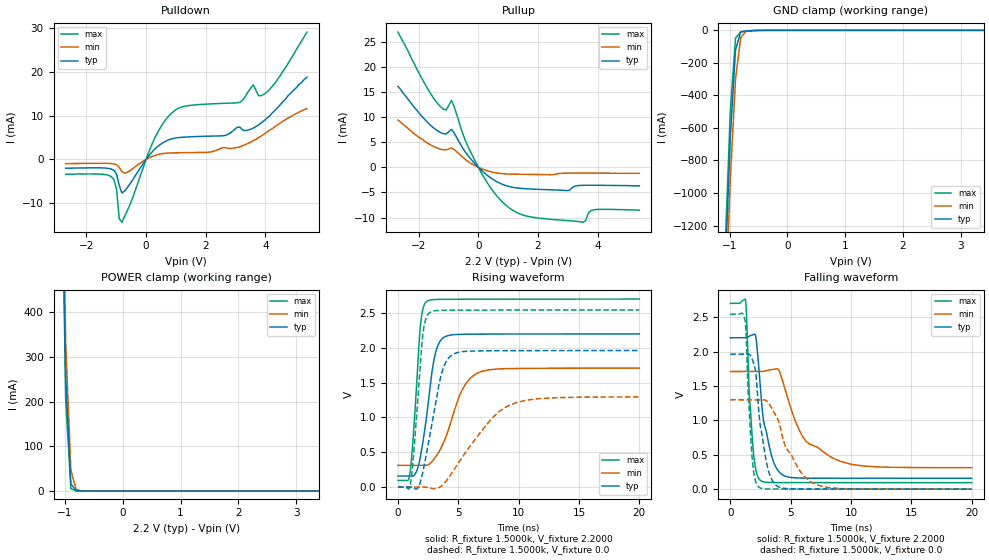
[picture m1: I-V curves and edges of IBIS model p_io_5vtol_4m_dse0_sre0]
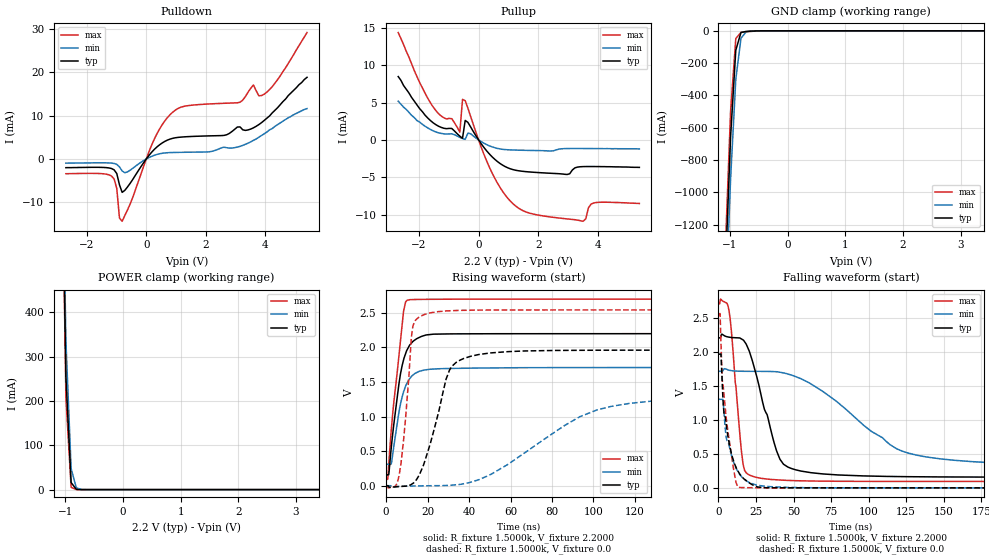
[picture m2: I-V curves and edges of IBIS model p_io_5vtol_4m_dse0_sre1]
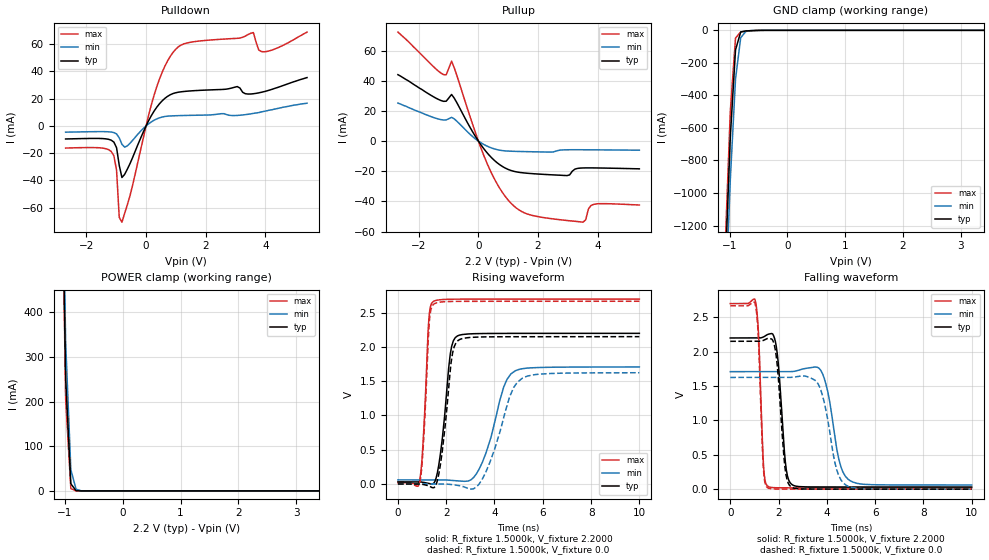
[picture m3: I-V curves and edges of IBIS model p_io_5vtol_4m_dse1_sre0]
| IBIS file nevis_64lqfp_derated.ibs generated by Daphne version: 2018.03.27
[IBIS Ver]   5.0
[Comment Char]   |_char
[File Name]   nevis_64lqfp_derated.ibs
[File Rev]   1
[Date]   Tue Nov  6 17:26:37 2018
[Source]   NXP Viper 2018.03.27
[Notes]
[Disclaimer] IMPORTANT NOTICE
  This information is provided on an AS IS basis and without warranty.
  IN NO EVENT SHALL NXP BE LIABLE FOR INCIDENTAL OR CONSEQUENTIAL
  DAMAGES ARISING FROM USE OF THIS INFORMATION. THIS DISCLAIMER OF
  WARRANTY EXTENDS TO THE USER OF THE INFORMATION, AND TO THEIR CUSTOMERS
  OR USERS OF PRODUCTS  AND IS IN LIEU OF ALL WARRANTIES WHETHER EXPRESS,
  IMPLIED, OR STATUTORY, INCLUDING IMPLIED WARRANTIES OF MERCHANTABILITY
  OR FITNESS FOR PARTICULAR PURPOSE.
  NXP does not represent or warrant that the information furnished
  hereunder is free of infringement of any third party patents,
  copyrights, trade secrets, or other intellectual property rights.
  NXP does not represent or warrant that the information is free of
  defect, or that it meets any particular standard, requirements or need
  of the user of the infomation or their customers.
  NXP reserves the right to change the information in this file
  without notice.
   http://www.nxp.com
[Copyright]   (C) Copyright NXP 2004 - 2018, All Rights Reserved.
|   NEVIS:64LQFP
[Component]   NEVIS:64LQFP
[Manufacturer]   NXP
[Package]
| variable   typ   min   max
R_pkg   0.18765   0.10323   0.21695
L_pkg   3.480e-09   3.024e-09   4.048e-09
C_pkg   4.328e-13   3.597e-13   5.462e-13
[Pin] signal_name   model_name   R_pin   L_pin   C_pin
1   TCK   p_io_5vtol_4m   0.20456   3.984e-09 4.456e-13
2   RESETB   p_vpp_5vtol_4m   0.10323   3.039e-09 5.462e-13
3   GPIOC0   p_io_5vtol_4m   0.18188   3.579e-09 5.125e-13
4   GPIOC1   p_io_5vtol_4m   0.17477   3.449e-09 4.197e-13
5   GPIOC2   p_io_5vtol_4m   0.17199   3.328e-09 4.057e-13
6   GPIOF8   p_io_5vtol_4m   0.1723   3.305e-09 3.675e-13
7   GPIOC3   p_io_5vtol_4m   0.17684   3.425e-09 4.342e-13
8   GPIOC4   p_io_5vtol_4m   0.17579   3.259e-09 3.771e-13
9   GPIOA7   p_io_5vtol_4m   0.1766   3.270e-09 3.648e-13
10   GPIOA6   p_io_5vtol_4m   0.17469   3.370e-09 3.597e-13
11   GPIOA5   p_io_5vtol_4m   0.17299   3.312e-09 3.848e-13
12   GPIOA4   p_io_5vtol_4m   0.17384   3.353e-09 4.083e-13
13   GPIOA0   p_io_5vtol_4m   0.17737   3.491e-09 4.216e-13
14   GPIOA1   p_io_5vtol_4m   0.18461   3.630e-09 4.562e-13
15   GPIOA2   p_io_5vtol_4m   0.19478   3.814e-09 5.013e-13
16   GPIOA3   p_io_5vtol_4m   0.20733   4.048e-09 4.586e-13
17   GPIOB7   p_io_5vtol_4m   0.20924   3.983e-09 4.401e-13
18   GPIOC5   p_io_5vtol_4m   0.10594   3.024e-09 5.247e-13
19   GPIOB6   p_io_5vtol_4m   0.19031   3.559e-09 4.944e-13
20   GPIOB5   p_io_5vtol_4m   0.18832   3.408e-09 4.217e-13
21   GPIOB4   p_io_5vtol_4m   0.19481   3.097e-09 4.139e-13
22   VDDA   POWER   NA   NA   NA
23   VSSA   GND   NA   NA   NA
24   GPIOB0   p_io_5vtol_4m   0.20499   3.148e-09 4.021e-13
25   GPIOB1   p_io_5vtol_4m   0.20867   3.139e-09 4.022e-13
26   VDD   POWER   NA   NA   NA
27   GPIOB2   p_io_5vtol_4m   0.21695   3.397e-09 3.938e-13
28   GPIOB3   p_io_5vtol_4m   0.20181   3.179e-09 4.053e-13
29   VDD33   POWER   NA   NA   NA
30   VSS   GND   NA   NA   NA
31   GPIOC6   p_io_5vtol_4m   0.20223   3.559e-09 4.815e-13
32   GPIOC7   p_io_5vtol_4m   0.20941   3.890e-09 4.421e-13
33   GPIOC8   p_io_5vtol_4m   0.20238   3.900e-09 4.381e-13
34   GPIOC9   p_io_5vtol_4m   0.18996   3.674e-09 4.850e-13
35   GPIOC10   p_io_5vtol_4m   0.18024   3.492e-09 4.400e-13
36   GPIOF0   p_io_5vtol_4m   0.17364   3.367e-09 3.978e-13
37   GPIOC11   p_io_5vtol_4m   0.17763   3.335e-09 3.915e-13
38   GPIOC12   p_io_5vtol_4m   0.17471   3.255e-09 3.726e-13
39   GPIOF2   p_io_5vtol_4m   0.17479   3.285e-09 3.730e-13
40   GPIOF3   p_io_5vtol_4m   0.17558   3.122e-09 3.751e-13
41   GPIOF4   p_io_5vtol_4m   0.1783   3.099e-09 3.845e-13
42   GPIOF5   p_io_5vtol_4m   0.18425   3.161e-09 4.158e-13
43   VSS   GND   NA   NA   NA
44   VDD33   POWER   NA   NA   NA
45   GPIOE0   p_io_5vtol_4m   0.18986   3.116e-09 4.169e-13
46   GPIOE1   p_io_5vtol_4m   0.19417   3.542e-09 4.935e-13
47   GPIOE2   p_io_5vtol_4m   0.19022   3.627e-09 4.739e-13
48   GPIOE3   p_io_5vtol_4m   0.20246   3.876e-09 4.382e-13
49   GPIOC13   p_io_5vtol_4m   0.20528   4.014e-09 4.475e-13
50   GPIOF1   p_io_5vtol_4m   0.1965   3.833e-09 4.884e-13
51   GPIOE4   p_io_5vtol_4m   0.2004   3.843e-09 4.592e-13
52   GPIOE5   p_io_5vtol_4m   0.19457   3.717e-09 4.386e-13
53   GPIOE6   p_io_5vtol_4m   0.19219   3.582e-09 4.273e-13
54   GPIOE7   p_io_5vtol_4m   0.19237   3.536e-09 3.947e-13
55   GPIOC14   p_io_5vtol_4m   0.19532   3.570e-09 3.956e-13
56   GPIOC15   p_io_5vtol_4m   0.19877   3.342e-09 3.979e-13
57   VDD   POWER   NA   NA   NA
58   GPIOF6   p_io_5vtol_4m   0.20225   3.248e-09 4.630e-13
59   GPIOF7   p_io_5vtol_4m   0.1991   3.203e-09 3.918e-13
60   VDD33   POWER   NA   NA   NA
61   VSS   GND   NA   NA   NA
62   TDO   p_io_5vtol_4m   0.19991   3.386e-09 5.235e-13
63   TMS   p_io_5vtol_4m   0.20172   3.751e-09 5.036e-13
64   TDI   p_io_5vtol_4m   0.21043   4.005e-09 4.589e-13
65   NC   NC   NA   NA   NA
[Pin Mapping]   pulldown_ref   pullup_ref
1   NC   NC
2   NC   NC
3   NC   NC
4   NC   NC
5   NC   NC
6   NC   NC
7   NC   NC
8   NC   NC
9   NC   NC
10   NC   NC
11   NC   NC
12   NC   NC
13   NC   NC
14   NC   NC
15   NC   NC
16   NC   NC
17   NC   NC
18   NC   NC
19   NC   NC
20   NC   NC
21   NC   NC
22   NC   VDDA
23   VSSA   NC
24   NC   NC
25   NC   NC
26   NC   VDD
27   NC   NC
28   NC   NC
29   NC   VDD33
30   VSS   NC
31   NC   NC
32   NC   NC
33   NC   NC
34   NC   NC
35   NC   NC
36   NC   NC
37   NC   NC
38   NC   NC
39   NC   NC
40   NC   NC
41   NC   NC
42   NC   NC
43   VSS   NC
44   NC   VDD33
45   NC   NC
46   NC   NC
47   NC   NC
48   NC   NC
49   NC   NC
50   NC   NC
51   NC   NC
52   NC   NC
53   NC   NC
54   NC   NC
55   NC   NC
56   NC   NC
57   NC   VDD
58   NC   NC
59   NC   NC
60   NC   VDD33
61   VSS   NC
62   NC   NC
63   NC   NC
64   NC   NC
65   NC   NC
|*   Model Selector   *
[Model Selector] p_io_5vtol_4m
p_io_5vtol_4m_dse1_sre0   io, full drive mode without slew rate
p_io_5vtol_4m_dse1_sre1   io, full drive mode with slew rate
p_io_5vtol_4m_dse0_sre0   io, low drive mode without slew rate
p_io_5vtol_4m_dse0_sre1   io, low drive mode with slew rate
| End [Component] NEVIS:64LQFP
| Models and submodels in the file (5): p_io_5vtol_4m_dse0_sre0 (I/O), p_io_5vtol_4m_dse0_sre1 (I/O), p_io_5vtol_4m_dse1_sre0 (I/O), p_io_5vtol_4m_dse1_sre1 (I/O), p_vpp_5vtol_4m (I/O_open_drain)
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[Model] p_io_5vtol_4m_dse0_sre0
|   Model p_io_5vtol_4m_dse0_sre0
| Library cells for typ/min/max conditions are connected as defined below:
|  pad - External Pad
|  ipp_do - Core Input
|  ipp_obe - Output Buffer Enable
|  esd_boost - vdd_s_3v
|  esd_bus - vdd_s_3v
|  ipp_ame - vss_s_lv
|  ipp_dse - vss_s_lv
|  ipp_ina40a_5vtol - NC
|  ipp_ina40b_5vtol - NC
|  ipp_ina_5vtol - NC
|  ipp_ina_mux_3v - NC
|  ipp_ind - NC
|  ipp_ind_3v - NC
|  ipp_pue - vss_s_lv
|  ipp_sre - vss_s_lv
|  tie_3v - vdd_s_3v
|  tie_hi - vdd_s_lv
|  vbuf_3v - vdd_s_3v
|  vdd_bulk_lv - vdd_s_lv
|  vdd_s_3v - vdd_s_3v
|  vdd_s_lv - vdd_s_lv
|  vss_bulk - vss_s_3v
|  vss_s_3v - vss_s_3v
|  vss_s_lv - vss_s_lv
| All other pins connected to ground
Model_type I/O
Polarity   Non-Inverting
Enable   Active-High
Vinl =   0.7700V
Vinh =   1.5400V
Vmeas =  1.1000V
Cref =   25.0000pF
Rref =   1.0000k
Vref =   0.0V
C_comp   2.5897pF   2.5141pF   2.6932pF
[Temperature Range]   25.0000   0.1250k   -40.0000
[Voltage Range]   2.2000V   1.7100V   2.7000V
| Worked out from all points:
|   slope of the pulldown table from 0 to 0.33 V, typ, clamps not added: 128 ohm
|   slope of the pullup table from 0 to 0.33 V, typ, clamps not added: 190 ohm
|   GND clamp passes 1 mA (typ) near -0.56 V on its own axis
|   POWER clamp passes 1 mA (typ) near -0.81 V on its own axis
|   rising waveform, R_fixture 1.5000k, V_fixture 2.2000: 20-80 % time 947ps typ, 1.78ns min, 566ps max; typ from 0.156 V to 2.2 V
|   rising waveform, R_fixture 1.5000k, V_fixture 0.0: 20-80 % time 1.26ns typ, 3.4ns min, 656ps max; typ from 0 V to 1.96 V
|   falling waveform, R_fixture 1.5000k, V_fixture 2.2000: 20-80 % time 953ps typ, 2.78ns min, 464ps max; typ from 2.2 V to 0.158 V
|   falling waveform, R_fixture 1.5000k, V_fixture 0.0: 20-80 % time 819ps typ, 1.91ns min, 430ps max; typ from 1.96 V to 0.001 V
[Pulldown]
|Voltage   I(typ)   I(min)   I(max)
-2.7V     -2mA       -960uA     -3.39mA
-1.17V    -2.19mA    -943uA     -3.913mA
-990mV    -3.359mA   -1.244mA   -6.804mA
-900mV    -5.941mA   -1.821mA   -13.58mA
-810mV    -7.677mA   -2.75mA    -14.34mA
270mV     2.201mA    843.7uA    4.568mA
810mV     4.605mA    1.475mA    10.28mA
3.15V     7.385mA    2.91mA     13.07mA
3.6V      7.17mA     4.3mA      17.03mA
3.78V     7.91mA     5mA        14.56mA
3.96V     8.86mA     5.8mA      14.91mA
5.4V      18.8mA     11.6mA     29.1mA
[Pullup]
|Voltage   I(typ)   I(min)   I(max)
-2.7V     16.1mA     9.4mA      26.9mA
-1.44V    7.55mA     3.98mA     13.23mA
-1.08V    6.637mA    3.488mA    11.41mA
-900mV    7.558mA    3.848mA    13.31mA
-450mV    3.121mA    1.623mA    5.492mA
90mV      -525.5uA   -231.9uA   -998.2uA
540mV     -2.585mA   -1.04mA    -5.11mA
1.08V     -3.888mA   -1.337mA   -8.259mA
2.97V     -4.634mA   -1.154mA   -10.59mA
3.51V     -3.575mA   -1.148mA   -10.91mA
3.87V     -3.565mA   -1.16mA    -8.446mA
5.4V      -3.68mA    -1.2mA     -8.52mA
[GND_clamp]
|Voltage   I(typ)   I(min)   I(max)
-2.7V     -20.35A    -20.38A    -20.37A
-1.08V    -1.486A    -1.737A    -1.339A
-990mV    -654.8mA   -915.7mA   -496.6mA
-900mV    -120.3mA   -300.6mA   -47.98mA
-810mV    -10.43mA   -45.61mA   -9.206mA
-720mV    -3.577mA   -6.172mA   -6.342mA
-540mV    -682.6uA   -563.7uA   -1.265mA
5.4V      0A         0A         0A
[POWER_clamp]
|Voltage   I(typ)   I(min)   I(max)
-2.7V     20.23A     19.96A     20.45A
-1.08V    950.5mA    990.2mA    948mA
-990mV    252.7mA    333.8mA    206.6mA
-900mV    16.05mA    47.59mA    5.278mA
-810mV    508.3uA    3.841mA    61.17uA
-720mV    15.33uA    281.3uA    694.4nA
-630mV    461.8nA    20.43uA    7.955nA
5.4V      0A         0A         0A
[Ramp]
| variable   typ   min   max
dV/dt_r  0.1310/0.6099n   41.9192m/0.9827n   0.3059/0.4620n
dV/dt_f  0.1585/0.2908n   47.3400m/0.4162n   0.3794/0.2202n
R_load = 50.0000
[Rising Waveform]
R_fixture= 1.5000k
V_fixture= 2.2000
V_fixture_min= 1.7100
V_fixture_max= 2.7000
|time   V(typ)   V(min)   V(max)
0s        156.3mV    309.1mV    94.08mV
1.008ns   156.1mV    309mV      214.5mV
1.223ns   156.9mV    309.1mV    604.9mV
1.884ns   453.4mV    309.7mV    2.358V
2.357ns   988.2mV    310.8mV    2.661V
3.11ns    1.925V     428.6mV    2.692V
4.041ns   2.17V      748mV      2.696V
5.622ns   2.194V     1.484V     2.697V
7.005ns   2.196V     1.663V     2.697V
20ns      2.198V     1.707V     2.699V
[Rising Waveform]
R_fixture= 1.5000k
V_fixture= 0.0
V_fixture_min= 0.0
V_fixture_max= 0.0
|time   V(typ)   V(min)   V(max)
0s        2.604nV    511.6nV    74.27pV
1.045ns   -1.902mV   -16.32uV   46.18mV
1.637ns   -19.77mV   562.3uV    1.241V
2.067ns   214.7mV    -137.8uV   2.196V
2.59ns    691.2mV    -13.1mV    2.501V
3.57ns    1.602V     7.719mV    2.537V
4.581ns   1.908V     230.7mV    2.539V
7.764ns   1.956V     982.8mV    2.541V
9.789ns   1.957V     1.211V     2.541V
20ns      1.959V     1.293V     2.542V
[Falling Waveform]
R_fixture= 1.5000k
V_fixture= 2.2000
V_fixture_min= 1.7100
V_fixture_max= 2.7000
|time   V(typ)   V(min)   V(max)
0s        2.2V       1.71V      2.7V
1.266ns   2.199V     1.71V      2.746V
1.857ns   2.244V     1.71V      666.2mV
2.139ns   2.193V     1.71V      267.4mV
2.491ns   1.482V     1.709V     127.5mV
3.471ns   456.6mV    1.739V     97.48mV
4.547ns   189.1mV    1.449V     96.53mV
6.025ns   161.2mV    756.7mV    96.23mV
8.664ns   159.3mV    438.4mV    95.93mV
20ns      158mV      313.1mV    95.07mV
[Falling Waveform]
R_fixture= 1.5000k
V_fixture= 0.0
V_fixture_min= 0.0
V_fixture_max= 0.0
|time   V(typ)   V(min)   V(max)
0s        1.962V     1.3V       2.544V
1.23ns    1.961V     1.299V     2.448V
1.507ns   1.965V     1.299V     1.307V
1.821ns   1.888V     1.299V     441mV
2.08ns    1.736V     1.299V     125.6mV
2.34ns    1.185V     1.299V     33.41mV
3.172ns   261.8mV    1.254V     3.37mV
4.045ns   30.97mV    963.9mV    2.355mV
7.029ns   2.701mV    73.09mV    1.814mV
20ns      1.37mV     2.257mV    877.9uV
[Model] p_io_5vtol_4m_dse0_sre1
|   Model p_io_5vtol_4m_dse0_sre1
| Library cells for typ/min/max conditions are connected as defined below:
|  pad - External Pad
|  ipp_do - Core Input
|  ipp_obe - Output Buffer Enable
|  esd_boost - vdd_s_3v
|  esd_bus - vdd_s_3v
|  ipp_ame - vss_s_lv
|  ipp_dse - vss_s_lv
|  ipp_ina40a_5vtol - NC
|  ipp_ina40b_5vtol - NC
|  ipp_ina_5vtol - NC
|  ipp_ina_mux_3v - NC
|  ipp_ind - NC
|  ipp_ind_3v - NC
|  ipp_pue - vss_s_lv
|  ipp_sre - vdd_s_lv
|  tie_3v - vdd_s_3v
|  tie_hi - vdd_s_lv
|  vbuf_3v - vdd_s_3v
|  vdd_bulk_lv - vdd_s_lv
|  vdd_s_3v - vdd_s_3v
|  vdd_s_lv - vdd_s_lv
|  vss_bulk - vss_s_3v
|  vss_s_3v - vss_s_3v
|  vss_s_lv - vss_s_lv
| All other pins connected to ground
Model_type I/O
Polarity   Non-Inverting
Enable   Active-High
Vinl =   0.7700V
Vinh =   1.5400V
Vmeas =  1.1000V
Cref =   25.0000pF
Rref =   1.0000k
Vref =   0.0V
C_comp   2.5897pF   2.5141pF   2.6932pF
[Temperature Range]   25.0000   0.1250k   -40.0000
[Voltage Range]   2.2000V   1.7100V   2.7000V
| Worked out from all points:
|   slope of the pulldown table from 0 to 0.33 V, typ, clamps not added: 128 ohm
|   slope of the pullup table from 0 to 0.33 V, typ, clamps not added: 190 ohm
|   GND clamp passes 1 mA (typ) near -0.56 V on its own axis
|   POWER clamp passes 1 mA (typ) near -0.81 V on its own axis
|   rising waveform, R_fixture 1.5000k, V_fixture 2.2000: 20-80 % time 5.65ns typ, 5.46ns min, 5.16ns max; typ from 0.156 V to 2.2 V
|   rising waveform, R_fixture 1.5000k, V_fixture 0.0: 20-80 % time 10.2ns typ, 40.8ns min, 4.04ns max; typ from 0 V to 1.96 V
|   falling waveform, R_fixture 1.5000k, V_fixture 2.2000: 20-80 % time 14.9ns typ, 48.1ns min, 5.86ns max; typ from 2.2 V to 0.157 V
|   falling waveform, R_fixture 1.5000k, V_fixture 0.0: 20-80 % time 7.69ns typ, 8.52ns min, 6.7ns max; typ from 1.96 V to 0 V
[Pulldown]
|Voltage   I(typ)   I(min)   I(max)
-2.7V     -2mA       -960uA     -3.39mA
-1.17V    -2.19mA    -943uA     -3.913mA
-990mV    -3.359mA   -1.244mA   -6.804mA
-900mV    -5.941mA   -1.821mA   -13.58mA
-810mV    -7.677mA   -2.75mA    -14.34mA
270mV     2.201mA    843.6uA    4.568mA
810mV     4.605mA    1.475mA    10.28mA
3.15V     7.385mA    2.91mA     13.07mA
3.6V      7.17mA     4.3mA      17.03mA
3.78V     7.91mA     5mA        14.56mA
3.96V     8.86mA     5.8mA      14.91mA
5.4V      18.8mA     11.6mA     29.1mA
[Pullup]
|Voltage   I(typ)   I(min)   I(max)
-2.7V     8.5mA      5.2mA      14.4mA
-1.35V    1.85mA     960uA      3.54mA
-630mV    503.1uA    337.6uA    1.039mA
-540mV    232uA      184.5uA    5.441mA
-450mV    2.62mA     76.25uA    5.267mA
-270mV    1.759mA    833.9uA    3.181mA
450mV     -2.247mA   -924uA     -4.401mA
1.35V     -4.138mA   -1.371mA   -9.168mA
2.97V     -4.634mA   -1.154mA   -10.59mA
3.51V     -3.575mA   -1.148mA   -10.91mA
3.87V     -3.565mA   -1.16mA    -8.446mA
5.4V      -3.68mA    -1.2mA     -8.52mA
[GND_clamp]
|Voltage   I(typ)   I(min)   I(max)
-2.7V     -20.35A    -20.38A    -20.37A
-1.08V    -1.486A    -1.737A    -1.339A
-990mV    -654.8mA   -915.7mA   -496.6mA
-900mV    -120.3mA   -300.6mA   -47.98mA
-810mV    -10.43mA   -45.61mA   -9.206mA
-720mV    -3.577mA   -6.172mA   -6.342mA
-540mV    -682.6uA   -563.7uA   -1.265mA
5.4V      0A         0A         0A
[POWER_clamp]
|Voltage   I(typ)   I(min)   I(max)
-2.7V     20.23A     19.96A     20.45A
-1.08V    950.5mA    990.2mA    948mA
-990mV    252.7mA    333.8mA    206.6mA
-900mV    16.05mA    47.59mA    5.278mA
-810mV    508.3uA    3.841mA    61.17uA
-720mV    15.33uA    281.3uA    694.4nA
-630mV    461.8nA    20.43uA    7.955nA
5.4V      0A         0A         0A
[Ramp]
| variable   typ   min   max
dV/dt_r  0.1311/23.4035n   41.8663m/52.4404n   0.3060/12.8070n
dV/dt_f  0.1582/45.1695n   44.5644m/78.6097n   0.3795/25.2219n
R_load = 50.0000
[Rising Waveform]
R_fixture= 1.5000k
V_fixture= 2.2000
V_fixture_min= 1.7100
V_fixture_max= 2.7000
|time   V(typ)   V(min)   V(max)
0s        156.3mV    309.1mV    94.08mV
815.6ps   157.1mV    309.1mV    105.6mV
1.298ns   167.8mV    309.1mV    331.9mV
2.604ns   593.5mV    333.2mV    856.3mV
6.029ns   1.445V     1.038V     1.844V
7.679ns   1.734V     1.282V     2.341V
8.414ns   1.822V     1.361V     2.529V
10.15ns   1.968V     1.489V     2.684V
22.89ns   2.193V     1.688V     2.698V
250ns     2.2V       1.71V      2.7V
[Rising Waveform]
R_fixture= 1.5000k
V_fixture= 0.0
V_fixture_min= 0.0
V_fixture_max= 0.0
|time   V(typ)   V(min)   V(max)
0s        2.604nV    511.6nV    74.27pV
5.747ns   -13.5mV    -12mV      81.86mV
8.324ns   -9.099mV   -8.182mV   632.2mV
12.6ns    26.88mV    -4.742mV   2.258V
18.59ns   350.7mV    -2.482mV   2.479V
30.52ns   1.672V     3.915mV    2.532V
40.3ns    1.869V     45.21mV    2.54V
93.45ns   1.96V      998.7mV    2.543V
108.8ns   1.961V     1.149V     2.544V
250ns     1.962V     1.298V     2.544V
[Falling Waveform]
R_fixture= 1.5000k
V_fixture= 2.2000
V_fixture_min= 1.7100
V_fixture_max= 2.7000
|time   V(typ)   V(min)   V(max)
0s        2.2V       1.71V      2.7V
6.944ns   2.212V     1.727V     2.608V
8.52ns    2.207V     1.72V      2.32V
15.27ns   2.186V     1.711V     541.7mV
17.35ns   2.146V     1.711V     258.9mV
20.57ns   2.003V     1.71V      188.7mV
38.71ns   541.7mV    1.704V     117.1mV
48.84ns   281.9mV    1.654V     106.5mV
126.3ns   163.9mV    510.7mV    94.31mV
250ns     156.6mV    328.6mV    94.08mV
[Falling Waveform]
R_fixture= 1.5000k
V_fixture= 0.0
V_fixture_min= 0.0
V_fixture_max= 0.0
|time   V(typ)   V(min)   V(max)
0s        1.962V     1.299V     2.544V
1.008ns   1.962V     1.299V     2.55V
1.612ns   1.955V     1.299V     2.128V
2.553ns   1.492V     1.3V       1.576V
3.481ns   1.132V     1.164V     1.404V
4.807ns   982mV      800.2mV    1.092V
8.792ns   484.8mV    465.6mV    459.7mV
12.95ns   246mV      239.2mV    12.26mV
30.99ns   2.45mV     24.33mV    945.8uV
250ns     336.6nV    50.98uV    -9.618nV
[Model] p_io_5vtol_4m_dse1_sre0
|   Model p_io_5vtol_4m_dse1_sre0
| Library cells for typ/min/max conditions are connected as defined below:
|  pad - External Pad
|  ipp_do - Core Input
|  ipp_obe - Output Buffer Enable
|  esd_boost - vdd_s_3v
|  esd_bus - vdd_s_3v
|  ipp_ame - vss_s_lv
|  ipp_dse - vdd_s_lv
|  ipp_ina40a_5vtol - NC
|  ipp_ina40b_5vtol - NC
|  ipp_ina_5vtol - NC
|  ipp_ina_mux_3v - NC
|  ipp_ind - NC
|  ipp_ind_3v - NC
|  ipp_pue - vss_s_lv
|  ipp_sre - vss_s_lv
|  tie_3v - vdd_s_3v
|  tie_hi - vdd_s_lv
|  vbuf_3v - vdd_s_3v
|  vdd_bulk_lv - vdd_s_lv
|  vdd_s_3v - vdd_s_3v
|  vdd_s_lv - vdd_s_lv
|  vss_bulk - vss_s_3v
|  vss_s_3v - vss_s_3v
|  vss_s_lv - vss_s_lv
| All other pins connected to ground
Model_type I/O
Polarity   Non-Inverting
Enable   Active-High
Vinl =   0.7700V
Vinh =   1.5400V
Vmeas =  1.1000V
Cref =   25.0000pF
Rref =   1.0000k
Vref =   0.0V
C_comp   2.5897pF   2.5141pF   2.6932pF
[Temperature Range]   25.0000   0.1250k   -40.0000
[Voltage Range]   2.2000V   1.7100V   2.7000V
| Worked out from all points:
|   slope of the pulldown table from 0 to 0.33 V, typ, clamps not added: 25.7 ohm
|   slope of the pullup table from 0 to 0.33 V, typ, clamps not added: 38.3 ohm
|   GND clamp passes 1 mA (typ) near -0.56 V on its own axis
|   POWER clamp passes 1 mA (typ) near -0.81 V on its own axis
|   rising waveform, R_fixture 1.5000k, V_fixture 2.2000: 20-80 % time 357ps typ, 774ps min, 207ps max; typ from 0.031 V to 2.2 V
|   rising waveform, R_fixture 1.5000k, V_fixture 0.0: 20-80 % time 368ps typ, 842ps min, 213ps max; typ from 0 V to 2.15 V
|   falling waveform, R_fixture 1.5000k, V_fixture 2.2000: 20-80 % time 259ps typ, 472ps min, 164ps max; typ from 2.2 V to 0.032 V
|   falling waveform, R_fixture 1.5000k, V_fixture 0.0: 20-80 % time 266ps typ, 512ps min, 164ps max; typ from 2.15 V to 0.001 V
[Pulldown]
|Voltage   I(typ)   I(min)   I(max)
-2.7V     -9.58mA    -4.57mA    -16.24mA
-1.17V    -10.45mA   -4.486mA   -18.73mA
-990mV    -15.98mA   -5.899mA   -32.6mA
-900mV    -28.96mA   -8.728mA   -67.1mA
-810mV    -37.86mA   -13.49mA   -70.68mA
270mV     10.92mA    4.187mA    22.64mA
990mV     24.34mA    7.491mA    56.19mA
3.06V     28.9mA     7.71mA     64.33mA
3.6V      23.63mA    9.2mA      68.56mA
3.78V     24.28mA    9.8mA      55.81mA
4.05V     25.71mA    11.1mA     54.67mA
5.4V      35.5mA     16.7mA     68.9mA
[Pullup]
|Voltage   I(typ)   I(min)   I(max)
-2.7V     44mA       25.2mA     72.2mA
-1.17V    26.34mA    13.97mA    43.99mA
-1.08V    26.42mA    14.03mA    43.92mA
-900mV    30.88mA    15.71mA    53mA
360mV     -9.303mA   -3.93mA    -17.88mA
810mV     -16.87mA   -6.301mA   -34.14mA
1.35V     -20.64mA   -6.862mA   -45.44mA
2.97V     -22.84mA   -5.752mA   -52.58mA
3.51V     -17.79mA   -5.736mA   -53.71mA
3.69V     -17.74mA   -5.75mA    -45.02mA
3.87V     -17.76mA   -5.78mA    -41.87mA
5.4V      -18.37mA   -6.03mA    -42.34mA
[GND_clamp]
|Voltage   I(typ)   I(min)   I(max)
-2.7V     -20.35A    -20.38A    -20.37A
-1.08V    -1.486A    -1.737A    -1.339A
-990mV    -654.8mA   -915.7mA   -496.6mA
-900mV    -120.3mA   -300.6mA   -47.98mA
-810mV    -10.43mA   -45.61mA   -9.206mA
-720mV    -3.577mA   -6.172mA   -6.342mA
-540mV    -682.6uA   -563.7uA   -1.265mA
5.4V      0A         0A         0A
[POWER_clamp]
|Voltage   I(typ)   I(min)   I(max)
-2.7V     20.23A     19.96A     20.45A
-1.08V    950.5mA    990.2mA    948mA
-990mV    252.7mA    333.8mA    206.6mA
-900mV    16.05mA    47.59mA    5.278mA
-810mV    508.3uA    3.841mA    61.17uA
-720mV    15.33uA    281.3uA    694.4nA
-630mV    461.8nA    20.43uA    7.955nA
5.4V      0A         0A         0A
[Ramp]
| variable   typ   min   max
dV/dt_r  0.6013/0.6303n   0.2061/1.0273n   1.0878/0.3490n
dV/dt_f  0.7290/0.3945n   0.2308/0.5522n   1.2634/0.2266n
R_load = 50.0000
[Rising Waveform]
R_fixture= 1.5000k
V_fixture= 2.2000
V_fixture_min= 1.7100
V_fixture_max= 2.7000
|time   V(typ)   V(min)   V(max)
0s        31.17mV    60.02mV    18.84mV
919.5ps   30.78mV    60.01mV    91.53mV
1.282ns   8.226mV    60.09mV    2.413V
1.447ns   3.959mV    60.27mV    2.659V
1.758ns   435.1mV    60.48mV    2.69V
2.169ns   1.9V       54.09mV    2.697V
2.459ns   2.16V      45.47mV    2.698V
3.365ns   2.196V     217.8mV    2.699V
4.869ns   2.199V     1.655V     2.699V
10ns      2.199V     1.708V     2.7V
[Rising Waveform]
R_fixture= 1.5000k
V_fixture= 0.0
V_fixture_min= 0.0
V_fixture_max= 0.0
|time   V(typ)   V(min)   V(max)
0s        554.5pV    116.8nV    15.42pV
925ps     -422.4uV   -11.58uV   53.71mV
1.296ns   -31.52mV   76.09uV    2.353V
1.461ns   -54.01mV   295.3uV    2.619V
1.698ns   153.9mV    642.5uV    2.652V
2.196ns   1.759V     -7.306mV   2.665V
2.486ns   2.094V     -20.73mV   2.666V
3.477ns   2.147V     59.83mV    2.667V
5.162ns   2.15V      1.547V     2.667V
10ns      2.151V     1.624V     2.667V
[Falling Waveform]
R_fixture= 1.5000k
V_fixture= 2.2000
V_fixture_min= 1.7100
V_fixture_max= 2.7000
|time   V(typ)   V(min)   V(max)
0s        2.2V       1.71V      2.7V
1.054ns   2.2V       1.71V      2.712V
1.378ns   2.215V     1.71V      342.1mV
1.534ns   2.249V     1.71V      48.36mV
1.907ns   2.075V     1.71V      21.05mV
2.282ns   395.9mV    1.709V     19.8mV
2.523ns   76.4mV     1.711V     19.62mV
3.755ns   32.34mV    1.726V     19.35mV
4.981ns   31.9mV     120.2mV    19.29mV
10ns      31.69mV    61.08mV    19.18mV
[Falling Waveform]
R_fixture= 1.5000k
V_fixture= 0.0
V_fixture_min= 0.0
V_fixture_max= 0.0
|time   V(typ)   V(min)   V(max)
0s        2.151V     1.626V     2.668V
1.036ns   2.151V     1.626V     2.693V
1.371ns   2.165V     1.626V     306.7mV
1.533ns   2.192V     1.626V     23.56mV
1.871ns   2.021V     1.626V     2.171mV
2.263ns   324.8mV    1.626V     928.9uV
2.513ns   34.93mV    1.627V     748.9uV
3.68ns    1.097mV    1.504V     496.2uV
4.791ns   728.7uV    59.37mV    439.6uV
10ns      501.2uV    942.9uV    324.1uV
